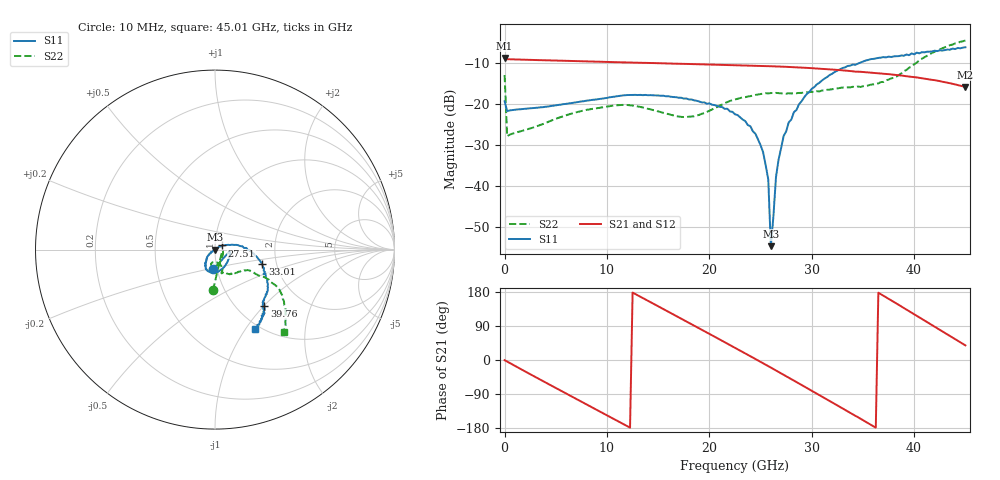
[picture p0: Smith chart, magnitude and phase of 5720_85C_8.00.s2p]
! Device:  ADRF5720
! Description: 0.5dB LSB GaAs MMIC 6-bit Digital Attenuator
! Frequency:  0.000009 -  40 GHz
! Ports:
!	RF1	= Port 1
!	RF2	= Port 2
! Vdd:  3.3 Volt
! Vss:  -3.3 Volt
! Control:  0/3.3 Volt
! State:  8.00 dB attenuation
! Data:  The device was measured using G-S-G Probes on a matrix board.
!  Data was collected using an calibrated 4 port network analyzer.
!  The reference plane for this measurement is at the launchers.
! Note:  Analog Devices supplies this data as a sample of measured data
!  for this product.  Your particular data for this product may vary.
!  Data was taken at 85 degrees C.
!  Analog Devices reserves the right to change this data at anytime.
# GHZ S DB R 45.0
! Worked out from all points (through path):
!   181 points, 10 MHz to 45.01 GHz, reference 45 ohm
!   highest |S21| = -8.72 dB at 10 MHz (marker M1); lowest = -15.8 dB at 45.01 GHz (marker M2)
!   group delay of S21, straight-line fit = 41.7 ps
!   lowest |S11| = -54.6 dB at 26.01 GHz (marker M3), VSWR 1.00, Z = 44.8 + j0.0178 ohm
!   |S11| at or under -10 dB: start of sweep to 34.61 GHz
!   |S22| runs from -27.8 to -4.5 dB; largest |S21 - S12| = 0.0017
!   S11 on the Smith chart (normalised r, x): 10 MHz: 0.96, -0.21; 27.51 GHz: 1.08, +0.05; 33.01 GHz: 1.68, -0.30; 39.76 GHz: 1.33, -1.00; 45.01 GHz: 0.95, -1.11
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0.01  -19.28 -94.4  -8.72 -0.5  -8.71 -0.5  -12.88 -92.8
0.26  -21.67 -7.1  -9.02 -4.0  -9.01 -4.0  -27.80 -11.9
4.26  -20.56 -38.1  -9.30 -63.0  -9.28 -62.9  -24.32 -51.7
7.76  -19.26 -62.1  -9.53 -113.7  -9.52 -113.6  -21.51 -76.7
11.51  -17.87 -85.8  -9.79 -167.7  -9.77 -167.6  -20.17 -97.0
15.26  -17.94 -106.3  -10.01 138.1  -9.99 138.2  -21.92 -105.0
19.01  -19.33 -119.2  -10.25 83.6  -10.23 83.7  -22.61 -78.5
22.76  -22.64 -129.4  -10.51 28.5  -10.50 28.7  -18.68 -69.7
24.01  -25.36 -138.2  -10.60 9.9  -10.58 10.2  -18.03 -71.8
25.26  -31.74 -149.0  -10.69 -8.7  -10.67 -8.4  -17.42 -73.6
25.76  -38.33 -153.8  -10.72 -16.2  -10.71 -16.0  -17.37 -73.9
26.01  -54.62 173.8  -10.74 -20.0  -10.73 -19.7  -17.27 -73.9
26.51  -37.83 40.9  -10.78 -27.6  -10.77 -27.3  -17.24 -73.6
27.26  -27.75 26.1  -10.86 -39.0  -10.84 -38.8  -17.34 -73.4
27.51  -26.60 29.7  -10.88 -42.8  -10.87 -42.5  -17.43 -72.4
28.26  -21.94 19.4  -10.97 -54.3  -10.96 -54.0  -17.28 -72.1
30.26  -15.81 3.3  -11.25 -85.1  -11.23 -84.9  -17.04 -66.9
33.01  -11.17 -17.2  -11.75 -127.9  -11.73 -127.7  -15.93 -59.4
37.76  -8.48 -41.4  -12.75 157.4  -12.73 157.7  -13.70 -34.4
39.76  -7.60 -48.7  -13.30 124.8  -13.28 125.2  -10.84 -30.5
42.26  -7.04 -53.5  -14.25 83.6  -14.23 84.0  -6.84 -34.3
45.01  -6.11 -63.1  -15.79 38.6  -15.76 38.9  -4.45 -50.2
